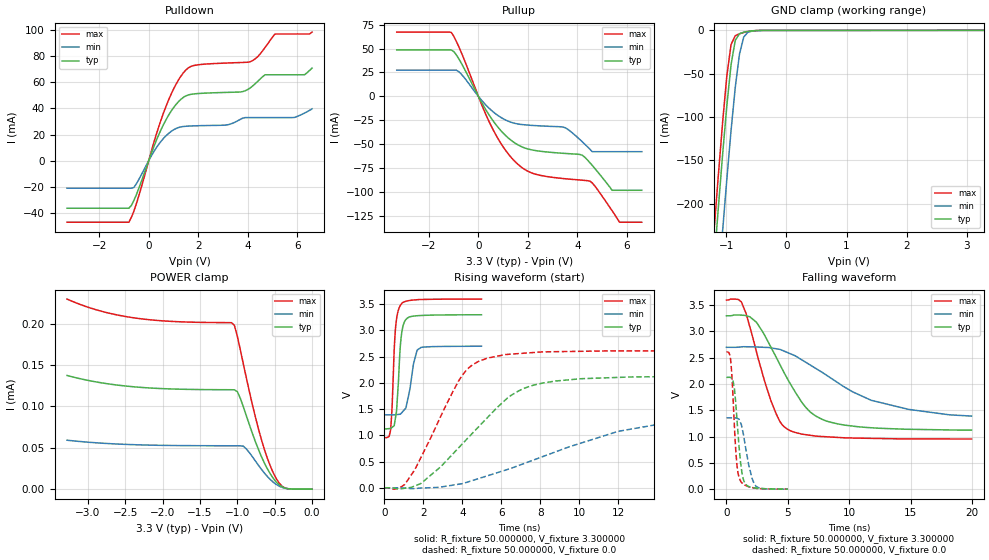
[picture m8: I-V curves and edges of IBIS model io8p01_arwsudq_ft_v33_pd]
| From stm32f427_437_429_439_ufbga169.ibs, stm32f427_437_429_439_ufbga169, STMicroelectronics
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|   Model io8p01_arwsudq_ft_v33_pd
[Model]  io8p01_arwsudq_ft_v33_pd
Model_type I/O
Polarity   Non-Inverting
Enable   Active-Low
Vinl =   0.990000V
Vinh =   2.310000V
Vmeas =  1.650000V
Cref =   50.000000pF
Rref =   100.000000M
Vref =   0.0V
C_comp   2.911600pF   2.826700pF   2.983100pF
[Temperature Range]   25.000000   0.125000k   -40.000000
[Pullup Reference]   3.300000V   2.700000V   3.600000V
[Pulldown Reference]   0.0V   0.0V   0.0V
[POWER Clamp Reference]   3.300000V   2.700000V   3.600000V
[GND Clamp Reference]   0.0V   0.0V   0.0V
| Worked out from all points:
|   slope of the pulldown table from 0 to 0.495 V, typ, clamps not added: 20.9 ohm
|   slope of the pullup table from 0 to 0.495 V, typ, clamps not added: 22.6 ohm
|   GND clamp passes 1 mA (typ) near -0.62 V on its own axis
|   rising waveform, R_fixture 50.000000, V_fixture 3.300000: 20-80 % time 220ps typ, 367ps min, 189ps max; typ from 1.12 V to 3.3 V
|   rising waveform, R_fixture 50.000000, V_fixture 0.0: 20-80 % time 3.34ns typ, 6.51ns min, 2.1ns max; typ from 0 V to 2.13 V
|   falling waveform, R_fixture 50.000000, V_fixture 3.300000: 20-80 % time 3.2ns typ, 6.17ns min, 2.04ns max; typ from 3.3 V to 1.12 V
|   falling waveform, R_fixture 50.000000, V_fixture 0.0: 20-80 % time 463ps typ, 671ps min, 372ps max; typ from 2.13 V to 0 V
[Pulldown]
|Voltage   I(typ)   I(min)   I(max)
-3.3V     -36.38mA   -21.07mA   -47.08mA
-800mV    -36.38mA   -21.07mA   -47.08mA
-600mV    -30.5mA    -20.54mA   -38.69mA
700mV     31.4mA     19.11mA    41.71mA
1.2V      45.15mA    25.37mA    61.75mA
1.6V      50.35mA    26.5mA     71.06mA
3.1V      52.27mA    27.26mA    74.75mA
4.1V      55.7mA     33.02mA    75.8mA
4.7V      65.79mA    33.02mA    86.63mA
5.1V      65.79mA    33.02mA    97.02mA
6.3V      65.87mA    36.5mA     97.02mA
6.6V      70.92mA    39.71mA    98.48mA
[Pullup]
|Voltage   I(typ)   I(min)   I(max)
-3.3V     48.52mA    27.43mA    67.13mA
-1.1V     48.52mA    27.43mA    66.86mA
-700mV    35.13mA    23.48mA    46.33mA
500mV     -22.07mA   -14mA      -30.03mA
1.5V      -49.1mA    -28.3mA    -68.56mA
2.2V      -56.04mA   -30.32mA   -80.35mA
3.5V      -59.53mA   -32.66mA   -85.92mA
4.2V      -61.45mA   -47.47mA   -87.46mA
4.5V      -69.1mA    -55.02mA   -88.4mA
5.4V      -98mA      -57.7mA    -119.3mA
5.7V      -98mA      -57.7mA    -131.3mA
6.6V      -98mA      -57.7mA    -131.3mA
[GND_clamp]
|Voltage   I(typ)   I(min)   I(max)
-3.3V     -2.32A     -2.397A    -2.297A
-1.2V     -266.4mA   -356.3mA   -229.4mA
-1.13V    -203.6mA   -293.1mA   -166.3mA
-1.06V    -143.2mA   -231.4mA   -106.2mA
-990mV    -86.95mA   -171.8mA   -52.65mA
-920mV    -39.66mA   -115.8mA   -16.37mA
-850mV    -11.5mA    -65.84mA   -6.125mA
-780mV    -3.846mA   -27.59mA   -3.894mA
-710mV    -2.102mA   -7.761mA   -2.396mA
-640mV    -1.159mA   -2.138mA   -1.234mA
-570mV    -535.1uA   -809uA     -490.2uA
3.28V     81.28uA    57.87uA    93.98uA
[POWER_clamp]
|Voltage   I(typ)   I(min)   I(max)
-3.28V    137.3uA    59.14uA    229.6uA
-2.36V    123.4uA    53.65uA    206.6uA
-1.08V    120.1uA    52.41uA    201.1uA
-1.04V    120uA      52.41uA    198uA
-1V       117.7uA    52.4uA     184.5uA
-920mV    99.46uA    51.91uA    151.2uA
-720mV    48.42uA    29.12uA    73.51uA
-600mV    24.82uA    15.47uA    37.72uA
-520mV    13.1uA     8.45uA     19.84uA
-440mV    5.058uA    3.61uA     7.276uA
-360mV    1.193uA    1.129uA    1.311uA
0V        0A         0A         0A
[Ramp]
| variable   typ   min   max
dV/dt_r  1.27692/3.33769n   0.80052/6.61392n   1.56696/2.09773n
dV/dt_f  1.30230/3.19734n   0.74358/6.21173n   1.58741/2.03810n
R_load = 50.000000
[Rising Waveform]
R_fixture= 50.000000
V_fixture= 3.300000
V_fixture_min= 2.700000
V_fixture_max= 3.600000
|time   V(typ)   V(min)   V(max)
0s        1.123V     1.391V     953.8mV
320.3ps   1.132V     1.39V      1.121V
390.4ps   1.152V     1.39V      1.529V
500.5ps   1.187V     1.39V      2.64V
620.6ps   1.466V     1.395V     3.218V
850.9ps   2.844V     1.417V     3.497V
1.101ns   3.208V     1.521V     3.555V
1.491ns   3.272V     2.365V     3.58V
1.682ns   3.28V      2.626V     3.585V
4.985ns   3.299V     2.699V     3.598V
[Rising Waveform]
R_fixture= 50.000000
V_fixture= 0.0
V_fixture_min= 0.0
V_fixture_max= 0.0
|time   V(typ)   V(min)   V(max)
0s        199.3uV    84.42uV    722.8uV
1.041ns   -9.231mV   -4.564mV   62.39mV
1.882ns   85.08mV    -4.083mV   582.9mV
3.884ns   790.7mV    71.98mV    2.08V
4.444ns   1.011V     129.4mV    2.321V
5.285ns   1.336V     227.8mV    2.471V
6.847ns   1.837V     417.9mV    2.557V
8.809ns   2.036V     687.4mV    2.595V
14.77ns   2.119V     1.255V     2.61V
19.94ns   2.127V     1.358V     2.611V
[Falling Waveform]
R_fixture= 50.000000
V_fixture= 3.300000
V_fixture_min= 2.700000
V_fixture_max= 3.600000
|time   V(typ)   V(min)   V(max)
0s        3.299V     2.699V     3.598V
1.241ns   3.31V      2.708V     3.548V
2.442ns   3.174V     2.705V     2.612V
3.604ns   2.708V     2.688V     1.692V
4.364ns   2.365V     2.658V     1.282V
5.045ns   2.065V     2.591V     1.13V
6.486ns   1.548V     2.409V     1.036V
8.328ns   1.282V     2.139V     994.4mV
11.77ns   1.169V     1.692V     966.6mV
19.94ns   1.123V     1.391V     953.8mV
[Falling Waveform]
R_fixture= 50.000000
V_fixture= 0.0
V_fixture_min= 0.0
V_fixture_max= 0.0
|time   V(typ)   V(min)   V(max)
0s        2.127V     1.358V     2.611V
340.3ps   2.124V     1.357V     2.46V
550.6ps   2.045V     1.357V     1.675V
680.7ps   1.831V     1.356V     1.042V
840.8ps   1.374V     1.349V     491.7mV
1.101ns   625.2mV    1.289V     179mV
1.451ns   139.9mV    943.6mV    84.04mV
1.822ns   49.55mV    451.2mV    44.41mV
2.362ns   22.36mV    67.85mV    18.47mV
4.985ns   199.3uV    84.42uV    722.8uV
